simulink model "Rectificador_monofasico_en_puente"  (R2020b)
settings: Solver=VariableStepAuto  StartTime=0.0  StopTime=200  RelTol=1e-3
libraries: powerlib x11

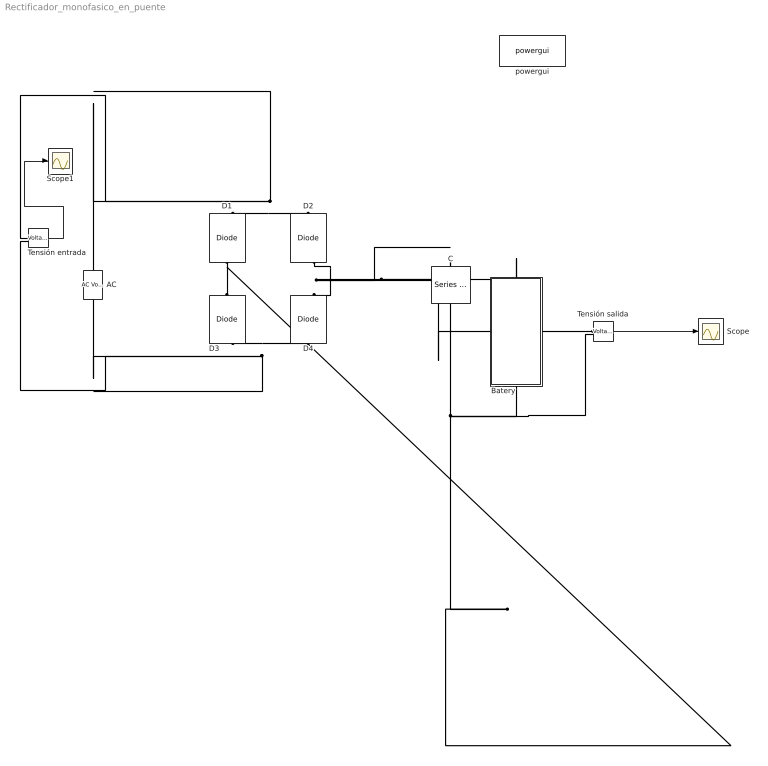
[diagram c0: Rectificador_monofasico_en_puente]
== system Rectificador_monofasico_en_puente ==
  "AC " : powerlib/Electrical Sources/AC Voltage Source  Amplitude=42  Phase=0  Frequency=50  SampleTime=0  Measurements=Voltage  BusType=swing  Pref=10e3  Qref=0  Qmin=-inf  Qmax=+inf
  Batery : Subsystem
  C : powerlib/Elements/Series RLC Branch  LConnTagsString=__new0  RConnTagsString=__new0  BranchType=C  Resistance=0  Inductance=1e-3  SetiL0=off  InitialCurrent=0  Capacitance=6600  Setx0=off  InitialVoltage=0  Measurements=None
  D{1..4} (4 alike) : powerlib/Power Electronics/Diode  Ron=0.001  Lon=0  Vf=0.8  IC=0  UseSnubber=0  Rs=500  Cs=250e-9  Measurements=on
  Scope : Scope
  Scope1 : Scope
  Tensión entrada : powerlib/Measurements/Voltage Measurement  PhasorSimulation=off  OutputType=Complex  PSBequivalent=0
  Tensión salida : powerlib/Measurements/Voltage Measurement  PhasorSimulation=off  OutputType=Complex  PSBequivalent=0
  powergui : powerlib/powergui  Priority=1  SimulationMode=Continuous  SampleTime=50e-6  frequency=60  Iterations=50  frequencyindice=50  Pbase=100e6  ErrMax=1e-4  UnitsV=kV  UnitsW=MW  buscounter=0  FunctionMessages=off  echomessages=off  EnableUseOfTLC=off  CurrentSourceSwitches=off  DisableSnubberDevices=off  DisableRonSwitches=off  DisableVfSwitches=off  DisplayEquations=off  AutomaticDiscreteSolvers=off  SolverType=Tustin/Backward Euler (TBE)  Interpol=off  ExternalGateDelay=off  methode=off  Ts=100  x0status=blocks  SPID=on  SwTol=0  HookPort=off  NonlinearTolerance=1e-4  nMaxIteration=100  ContinueOnMaxIteration=off  RestoreLinks=warning  ResistiveCurrentMeasurement=off  Frange=[0:2:500]  Ylog=off  Xlog=on  ShowGrid=off  save=off  variable=ZData  structure=0  ZoomFFT=off  StartTime=0.0  cycles=1  DisplayStyle=1  fundamental=60  FreqAxis=off  MaxFrequency=1000  frequencyindicesteady=1  RmsSteady=1  display=off
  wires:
  Tensión entrada/1 -> Scope1/1
  Tensión salida/1 -> Scope/1
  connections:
  D1/RConn1 -- "AC "/RConn1 -- Tensión entrada/LConn1 -- D2/LConn1
  D1/LConn1 -- Tensión salida/LConn2 -- Batery/LConn1 -- C/RConn1 -- D3/LConn1
  D4/LConn1 -- "AC "/LConn1 -- Tensión entrada/LConn2 -- D3/RConn1
  D2/RConn1 -- C/LConn1 -- Batery/RConn1 -- Tensión salida/LConn1 -- D4/RConn1

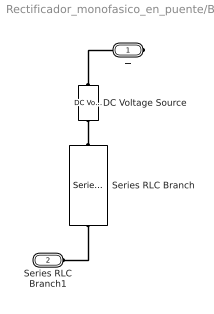
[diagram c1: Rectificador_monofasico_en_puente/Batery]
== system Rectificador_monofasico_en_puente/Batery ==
  DC Voltage Source : powerlib/Electrical Sources/DC Voltage Source  Amplitude=12  Measurements=Voltage
  Series RLC Branch : powerlib/Elements/Series RLC Branch  LConnTagsString=__new0  RConnTagsString=__new0  BranchType=R  Resistance=100  Inductance=1e-3  SetiL0=off  InitialCurrent=0  Capacitance=1e-6  Setx0=off  InitialVoltage=0  Measurements=None
  + : PMIOPort  Side=Right
  Series RLC Branch1 : PMIOPort  Port=2  Side=Left
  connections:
  Series RLC Branch/RConn1 -- DC Voltage Source/LConn1
  Series RLC Branch/LConn1 -- Series RLC Branch1/RConn1
  DC Voltage Source/RConn1 -- +/RConn1
